FUNCTION "MODI MACCHINA" : VOID
TITLE =MODI OPERATIVI MACCHINA
VERSION : 0.1

BEGIN
NETWORK
TITLE =MANUALE - JOG-REF - AUTOMATICO
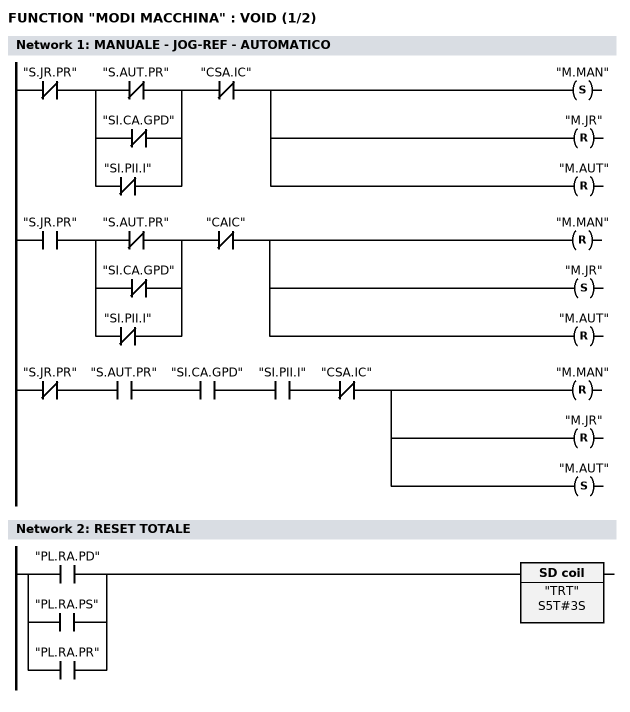
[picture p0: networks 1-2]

      UN    "S.JR.PR";
      U(    ;
      ON    "S.AUT.PR";
      ON    "SI.CA.GPD";
      ON    "SI.PII.I";
      )     ;
//-
      UN    "CSA.IC";
      S     "M.MAN";
      R     "M.JR";
      R     "M.AUT";
      U     "S.JR.PR";
      U(    ;
//-
      ON    "S.AUT.PR";
      ON    "SI.CA.GPD";
      ON    "SI.PII.I";
      )     ;
      UN    "CAIC";
      R     "M.MAN";

      S     "M.JR";
      R     "M.AUT";
      UN    "S.JR.PR";
      U     "S.AUT.PR";
      U     "SI.CA.GPD";
      U     "SI.PII.I";
      UN    "CSA.IC";
      R     "M.MAN";
      R     "M.JR";
      S     "M.AUT";

NETWORK
TITLE =RESET TOTALE

      O     "PL.RA.PD";
      O     "PL.RA.PS";
      O     "PL.RA.PR";
      L     S5T#3S;
      SE    "TRT";
NETWORK
TITLE =POSIZIONI MANIPOLATORI
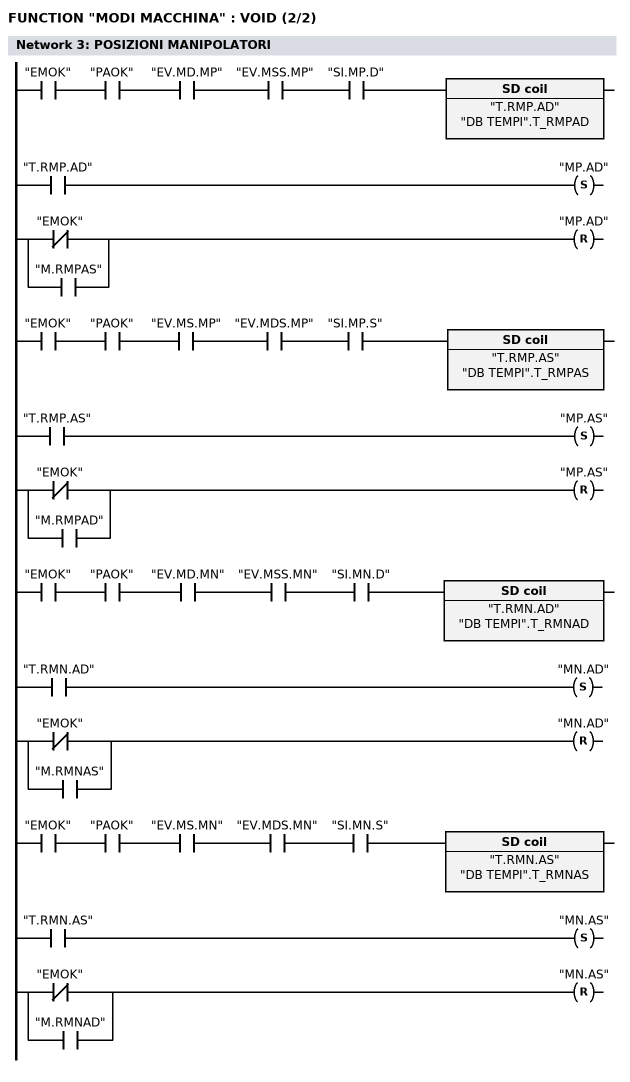
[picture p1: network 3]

      U     "EMOK";
      U     "PAOK";
      U     "EV.MD.MP";
      U     "EV.MSS.MP";
      U     "SI.MP.D";
      L     "DB TEMPI".T_RMPAD;
      SE    "T.RMP.AD";
      U     "T.RMP.AD";
      S     "MP.AD";
//----------------------
      ON    "EMOK";
      O     "M.RMPAS";
      R     "MP.AD";
//======================
      U     "EMOK";
      U     "PAOK";
      U     "EV.MS.MP";
      U     "EV.MDS.MP";
      U     "SI.MP.S";
      L     "DB TEMPI".T_RMPAS;
      SE    "T.RMP.AS";
      U     "T.RMP.AS";
      S     "MP.AS";
//----------------------
      ON    "EMOK";
      O     "M.RMPAD";
      R     "MP.AS";
//======================
      U     "EMOK";
      U     "PAOK";
      U     "EV.MD.MN";
      U     "EV.MSS.MN";
      U     "SI.MN.D";
      L     "DB TEMPI".T_RMNAD;
      SE    "T.RMN.AD";
      U     "T.RMN.AD";
      S     "MN.AD";
//----------------------
      ON    "EMOK";
      O     "M.RMNAS";
      R     "MN.AD";
//======================
      U     "EMOK";
      U     "PAOK";
      U     "EV.MS.MN";
      U     "EV.MDS.MN";
      U     "SI.MN.S";
      L     "DB TEMPI".T_RMNAS;
      SE    "T.RMN.AS";
      U     "T.RMN.AS";
      S     "MN.AS";
//----------------------
      ON    "EMOK";
      O     "M.RMNAD";
      R     "MN.AS";
END_FUNCTION

